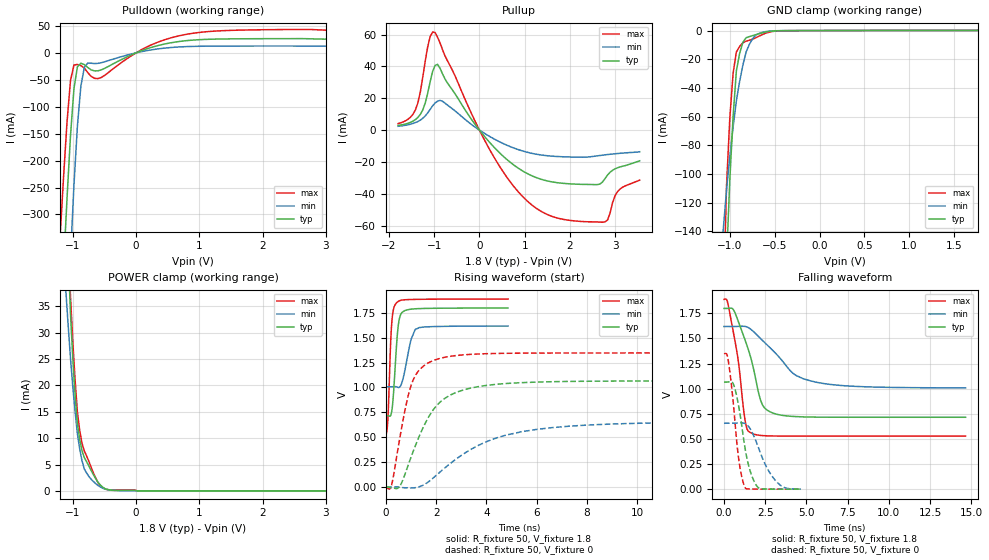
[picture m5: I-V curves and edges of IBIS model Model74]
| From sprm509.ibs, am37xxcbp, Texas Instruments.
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| Model based on original model for BQ18OMAPSMART1HYFBPBNOPM_SSBHV
|   Sub model NOPM_VS01L11_PD1_1P8
[model]   Model74
|[Input Load]   PD
|[Output Drive] SC01LB11
|Voltage   1.8V
|Mode   I/O
Model_type   I/O
Polarity   Non-Inverting
Enable   Active-Low
Vinl =  0.63
Vinh =  1.17
Cref =  15pF
Rref =  100.0000M
Vref =  0V
Vmeas =  0.9
C_comp   1.410688p   1.256095p   1.577871p
[Model Spec]
Vinl   0.63   0.567   0.6615
Vinh   1.17   1.053   1.2285
[Temperature Range]   25   125   -40
[Voltage Range]   1.8   1.62   1.89
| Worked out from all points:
|   slope of the pulldown table from 0 to 0.27 V, typ, clamps not added: 24.3 ohm
|   slope of the pullup table from 0 to 0.27 V, typ, clamps not added: 29.7 ohm
|   GND clamp passes 1 mA (typ) near -0.60 V on its own axis
|   POWER clamp passes 1 mA (typ) near -0.55 V on its own axis
|   rising waveform, R_fixture 50, V_fixture 1.8: 20-80 % time 175ps typ, 302ps min, 124ps max; typ from 0.715 V to 1.8 V
|   rising waveform, R_fixture 50, V_fixture 0: 20-80 % time 1.28ns typ, 2.76ns min, 685ps max; typ from 0 V to 1.06 V
|   falling waveform, R_fixture 50, V_fixture 1.8: 20-80 % time 1.08ns typ, 2.15ns min, 678ps max; typ from 1.8 V to 0.715 V
|   falling waveform, R_fixture 50, V_fixture 0: 20-80 % time 669ps typ, 1.08ns min, 497ps max; typ from 1.06 V to 0 V
[POWER_clamp]
-1.8V     362.5mA    191.4mA    412.8mA
-1.109V   56.75mA    37.73mA    60.5mA
-1.073V   44.66mA    31.25mA    47.93mA
-1.036V   33.51mA    25.07mA    36.73mA
-1V       25.06mA    19.75mA    28.2mA
-963.6mV  18.11mA    14.99mA    20.92mA
-927.3mV  12.68mA    10.81mA    14.88mA
-890.9mV  9.743mA    7.94mA     11.46mA
-818.2mV  6.308mA    4.161mA    7.567mA
-563.6mV  1.112mA    743.5uA    1.008mA
18.18mV   0A         0A         0A
3.6V      0A         0A         0A
[Pulldown]
-1.8V     -1.718A    -2.61A     -1.406A
-1.2V     -527.4mA   -844.5mA   -339.9mA
-1.145V   -396mA     -683.1mA   -229.1mA
-1.091V   -269mA     -526.7mA   -127.5mA
-1.036V   -153.6mA   -378.9mA   -51.17mA
-981.8mV  -66.33mA   -245.6mA   -22.67mA
-927.3mV  -26mA      -136.2mA   -21.54mA
-872.7mV  -19.34mA   -61.98mA   -23.69mA
-763.6mV  -27.2mA    -19.05mA   -36.72mA
-545.5mV  -31.39mA   -18.17mA   -45.46mA
872.7mV   23.46mA    11.88mA    35.92mA
3.545V    25.34mA    12.51mA    41.58mA
[Pullup]
-1.8V     2.903mA    2.423mA    4.112mA
-1.418V   6.595mA    4.711mA    12.64mA
-1.255V   12.69mA    7.42mA     33.24mA
-1.091V   30.4mA     13mA       58.69mA
-981.8mV  40.63mA    17.02mA    61.3mA
-818.2mV  35.38mA    18.12mA    50.59mA
272.7mV   -9.18mA    -4.728mA   -14.55mA
1.255V    -29.75mA   -15.09mA   -48.97mA
2.564V    -34.17mA   -16.31mA   -57.57mA
2.782V    -30.25mA   -15.5mA    -57.49mA
3.055V    -23.63mA   -14.68mA   -38.61mA
3.545V    -19.25mA   -13.56mA   -31.41mA
[GND_clamp]
-1.8V     -2.82A     -1.192A    -3.165A
-1.073V   -235.8mA   -138.4mA   -192.1mA
-1.036V   -159.6mA   -110.8mA   -107.6mA
-1V       -103.8mA   -87.86mA   -60.72mA
-963.6mV  -60.04mA   -67.3mA    -29.85mA
-927.3mV  -28.26mA   -49.1mA    -14.96mA
-890.9mV  -15.95mA   -35.5mA    -11.07mA
-854.5mV  -8.196mA   -24.09mA   -8.539mA
-818.2mV  -4.988mA   -14.87mA   -7.364mA
-709.1mV  -2.851mA   -3.095mA   -4.982mA
-563.6mV  -633.9uA   -437.8uA   -1.185mA
1.764V    107.4uA    58.81uA    171.2uA
[Ramp]
dV/dt_f  0.6514877/1.080487n   0.3682855/2.164736n   0.8179735/0.6799974n
dV/dt_r  0.6494217/1.282549n   0.3998341/2.786173n   0.8209353/0.686378n
R_load = 50
[Rising Waveform]
R_fixture = 50
V_fixture = 1.8
V_fixture_min = 1.62
V_fixture_max = 1.89
0s        715.1mV    1.007V     525.8mV
81ps      717.2mV    1.007V     717mV
180ps     716.1mV    1.007V     1.426V
234ps     770.1mV    1.007V     1.667V
396ps     1.337V     1.007V     1.844V
486ps     1.62V      999.5mV    1.864V
567ps     1.722V     1.011V     1.874V
999ps     1.786V     1.484V     1.883V
1.161ns   1.79V      1.582V     1.884V
4.86ns    1.798V     1.617V     1.888V
[Rising Waveform]
R_fixture = 50
V_fixture = 0
V_fixture_min = 0
V_fixture_max = 0
0s        161uV      101.7uV    -10.97mV
225ps     -10.1mV    -199.8uV   21.94mV
576ps     19.2mV     -3.806mV   530.7mV
846ps     193.3mV    -8.423mV   877.9mV
1.071ns   350.4mV    -10.07mV   1.07V
1.602ns   660mV      36.2mV     1.234V
2.088ns   836.7mV    136.4mV    1.288V
3.888ns   1.016V     442.4mV    1.338V
6.012ns   1.054V     578.9mV    1.345V
19.04ns   1.065V     654.3mV    1.346V
[Falling Waveform]
R_fixture = 50
V_fixture = 1.8
V_fixture_min = 1.62
V_fixture_max = 1.89
0s        1.798V     1.618V     1.888V
198ps     1.798V     1.619V     1.872V
585ps     1.782V     1.618V     1.548V
882ps     1.663V     1.62V      1.258V
1.269ns   1.489V     1.619V     695.4mV
1.602ns   1.321V     1.594V     562.9mV
2.349ns   834.1mV    1.478V     533mV
3.132ns   748.6mV    1.352V     528.9mV
5.661ns   716.6mV    1.062V     528.1mV
14.66ns   715.4mV    1.008V     528.1mV
[Falling Waveform]
R_fixture = 50
V_fixture = 0
V_fixture_min = 0
V_fixture_max = 0
0s        1.065V     655.7mV    1.347V
270ps     1.067V     656.1mV    1.268V
648ps     1.009V     656.3mV    706.1mV
936ps     783.7mV    659.5mV    250.5mV
1.278ns   407.9mV    653mV      16.97mV
1.593ns   178.4mV    599.2mV    1.815mV
2.07ns    16.69mV    422.4mV    228.9uV
2.619ns   1.52mV     208.8mV    25.62uV
3.267ns   335uV      61.33mV    3.219uV
4.671ns   50.74uV    1.646mV    422nV
